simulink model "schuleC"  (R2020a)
settings: Solver=FixedStepDiscrete  StartTime=0.0  StopTime=30  FixedStep=1  RelTol=1e-3  EnableMultiTasking=on

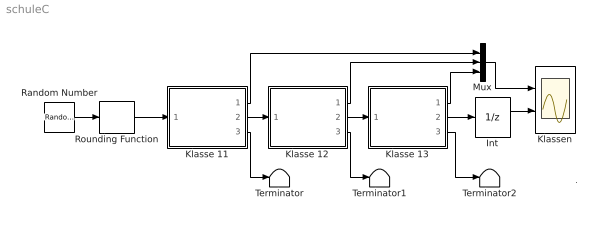
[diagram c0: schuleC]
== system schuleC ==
  note: .
  Int : UnitDelay  SampleTime=-1  HasFrameUpgradeWarning=on
  Klasse 11 : Subsystem  mask{x0=0, W=0.08, A=0.03}
      mask prompts: x0 "Anfangsstaerke"; W "Wiederholerrate"; A "Abbrecherrate"
  Klasse 12 : Subsystem  mask{x0=0, W=0.08, A=0.07}
      mask prompts: x0 "Anfangsstaerke"; W "Wiederholerrate"; A "Abbrecherrate"
  Klasse 13 : Subsystem  mask{x0=0, W=0.04, A=0.04}
      mask prompts: x0 "Anfangsstaerke"; W "Wiederholerrate"; A "Abbrecherrate"
  Klassen : Scope  NumInputPorts=2
  Mux : Mux  Inputs=3
  Random Number : RandomNumber  Mean=30  Variance=10  Seed=42  SampleTime=0
  Rounding Function : Rounding  Operator=round
  Terminator : Terminator
  Terminator1 : Terminator
  Terminator2 : Terminator
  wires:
  Klasse 11/2(versetzt) -> Klasse 12/1(neu)
  Klasse 12/2(versetzt) -> Klasse 13/1(neu)
  Klasse 13/2(versetzt) -> Int/1
  Mux/1 -> Klassen/1
  Klasse 11/1(Klassenstaerke) -> Mux/1
  Klasse 12/1(Klassenstaerke) -> Mux/2
  Random Number/1 -> Rounding Function/1
  Rounding Function/1 -> Klasse 11/1(neu)
  Int/1 -> Klassen/2
  Klasse 11/3(abgegangen) -> Terminator/1
  Klasse 12/3(abgegangen) -> Terminator1/1
  Klasse 13/3(abgegangen) -> Terminator2/1
  Klasse 13/1(Klassenstaerke) -> Mux/3

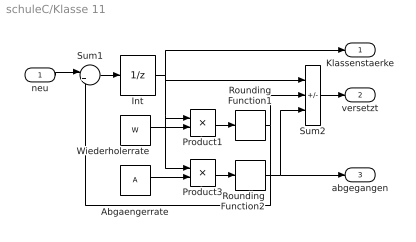
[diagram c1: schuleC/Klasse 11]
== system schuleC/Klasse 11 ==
  neu : Inport
  Abgaengerrate : Constant  Value=A
  Int : UnitDelay  InitialCondition=x0  SampleTime=-1  HasFrameUpgradeWarning=on
  Product1 : Product  InputSameDT=on  RndMeth=Zero  SaturateOnIntegerOverflow=on
  Product3 : Product  InputSameDT=on  RndMeth=Zero  SaturateOnIntegerOverflow=on
  Rounding Function1 : Rounding  Operator=round
  Rounding Function2 : Rounding  Operator=round
  Sum1 : Sum  Inputs=|++  InputSameDT=on  SaturateOnIntegerOverflow=on
  Sum2 : Sum  Inputs=+--  InputSameDT=on  SaturateOnIntegerOverflow=on
  Wiederholerrate : Constant  Value=W
  Klassenstaerke : Outport
  versetzt : Outport  Port=2
  abgegangen : Outport  Port=3
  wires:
  Sum1/1 -> Int/1
  Wiederholerrate/1 -> Product1/2
  Int/1 -> Klassenstaerke/1, Product1/1, Product3/1, Sum2/1
  Abgaengerrate/1 -> Product3/2
  Product1/1 -> Rounding Function1/1
  Product3/1 -> Rounding Function2/1
  neu/1 -> Sum1/1
  Sum2/1 -> versetzt/1
  Rounding Function1/1 -> Sum1/2, Sum2/2
  Rounding Function2/1 -> abgegangen/1, Sum2/3

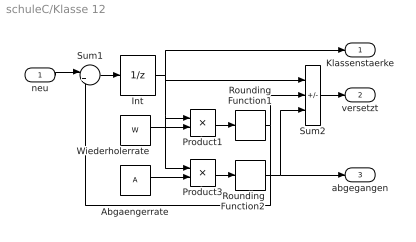
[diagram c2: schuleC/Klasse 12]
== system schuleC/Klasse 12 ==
  neu : Inport
  Abgaengerrate : Constant  Value=A
  Int : UnitDelay  InitialCondition=x0  SampleTime=-1  HasFrameUpgradeWarning=on
  Product1 : Product  InputSameDT=on  RndMeth=Zero  SaturateOnIntegerOverflow=on
  Product3 : Product  InputSameDT=on  RndMeth=Zero  SaturateOnIntegerOverflow=on
  Rounding Function1 : Rounding  Operator=round
  Rounding Function2 : Rounding  Operator=round
  Sum1 : Sum  Inputs=|++  InputSameDT=on  SaturateOnIntegerOverflow=on
  Sum2 : Sum  Inputs=+--  InputSameDT=on  SaturateOnIntegerOverflow=on
  Wiederholerrate : Constant  Value=W
  Klassenstaerke : Outport
  versetzt : Outport  Port=2
  abgegangen : Outport  Port=3
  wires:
  Rounding Function2/1 -> Sum2/3, abgegangen/1
  Rounding Function1/1 -> Sum2/2, Sum1/2
  Sum2/1 -> versetzt/1
  neu/1 -> Sum1/1
  Product3/1 -> Rounding Function2/1
  Product1/1 -> Rounding Function1/1
  Abgaengerrate/1 -> Product3/2
  Int/1 -> Sum2/1, Product3/1, Product1/1, Klassenstaerke/1
  Wiederholerrate/1 -> Product1/2
  Sum1/1 -> Int/1

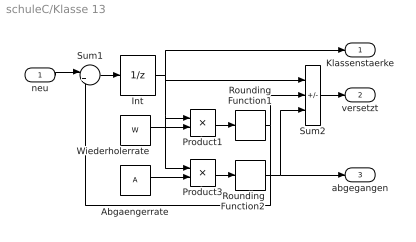
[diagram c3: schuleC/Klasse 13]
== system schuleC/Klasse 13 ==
  neu : Inport
  Abgaengerrate : Constant  Value=A
  Int : UnitDelay  InitialCondition=x0  SampleTime=-1  HasFrameUpgradeWarning=on
  Product1 : Product  InputSameDT=on  RndMeth=Zero  SaturateOnIntegerOverflow=on
  Product3 : Product  InputSameDT=on  RndMeth=Zero  SaturateOnIntegerOverflow=on
  Rounding Function1 : Rounding  Operator=round
  Rounding Function2 : Rounding  Operator=round
  Sum1 : Sum  Inputs=|++  InputSameDT=on  SaturateOnIntegerOverflow=on
  Sum2 : Sum  Inputs=+--  InputSameDT=on  SaturateOnIntegerOverflow=on
  Wiederholerrate : Constant  Value=W
  Klassenstaerke : Outport
  versetzt : Outport  Port=2
  abgegangen : Outport  Port=3
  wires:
  Sum1/1 -> Int/1
  Wiederholerrate/1 -> Product1/2
  Int/1 -> Klassenstaerke/1, Product1/1, Product3/1, Sum2/1
  Abgaengerrate/1 -> Product3/2
  Product1/1 -> Rounding Function1/1
  Product3/1 -> Rounding Function2/1
  neu/1 -> Sum1/1
  Sum2/1 -> versetzt/1
  Rounding Function1/1 -> Sum1/2, Sum2/2
  Rounding Function2/1 -> abgegangen/1, Sum2/3
